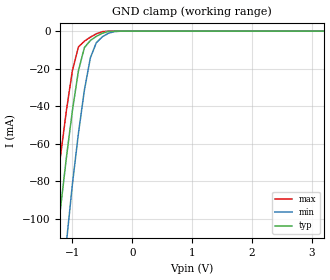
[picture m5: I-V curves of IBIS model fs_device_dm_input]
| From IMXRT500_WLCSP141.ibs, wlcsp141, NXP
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[Model] fs_device_dm_input
|   Model fs_device_dm_input
| Library cells for typ/min/max conditions are connected as defined below:
|  pad_usbdp - External Pad
|  d_dmpulldn - gnda
|  d_dppulldn - gnda
|  d_sw1_neg - gnda
|  d_sw1_pos - gnda
|  d_sw2_neg - gnda
|  d_sw2_pos - gnda
|  gnda - gnda
|  pad_usb_vss - pad_usb_vss
|  usb2_reg_tx_fs_hiz - vddd
|  usb2_reg_tx_hs_term - gnda
|  usb2_reg_tx_hs_xcvr - gnda
|  usb2_reg_tx_ls_en - gnda
|  usbphy_d2a_txhsactive - gnda
|  vddb - vddb
|  vddd - vddd
| All other pins connected to ground
Model_type Input
Vinl =   0.800V
Vinh =   2.000V
C_comp   2.8431pF   2.6338pF   3.0727pF
[Temperature Range]   27.0000   0.1250k   -40.0000
[Voltage Range]   3.1500V   3.0000V   3.3000V
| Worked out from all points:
|   GND clamp passes 1 mA (typ) near -0.49 V on its own axis
[GND_clamp]
|Voltage   I(typ)   I(min)   I(max)
-3.3V     -1.77A     -1.861A    -1.685A
-1.4V     -157.5mA   -242mA     -123.2mA
-1.3V     -124.5mA   -192mA     -93.92mA
-1.2V     -94.75mA   -149.4mA   -66.83mA
-1.1V     -67.24mA   -112.7mA   -42.19mA
-1V       -42.28mA   -81.53mA   -20.95mA
-900mV    -21.21mA   -54.56mA   -8.451mA
-800mV    -8.759mA   -31.44mA   -5.347mA
-700mV    -4.979mA   -14.22mA   -3.195mA
-600mV    -2.775mA   -6.133mA   -1.408mA
-200mV    -368.5nA   -34.12uA   -8.977nA
3.2V      34.24nA    35.64uA    32.08nA
